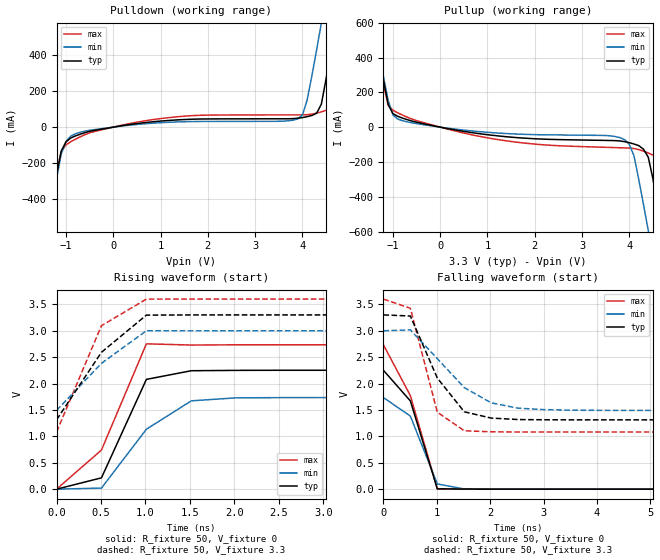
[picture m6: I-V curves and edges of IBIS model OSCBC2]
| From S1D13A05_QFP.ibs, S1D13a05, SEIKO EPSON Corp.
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[Model]   OSCBC2
Model_type Output
Polarity Non-Inverting
Vref=0
Vmeas=1.65
Rref=500
Cref=100pf
C_comp   5p   4p   6p
[Temperature Range] 25   85   -40
[Voltage Range]   3.3   3.0   3.6
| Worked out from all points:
|   slope of the pulldown table from 0 to 0.495 V, typ, clamps not added: 25.1 ohm
|   slope of the pullup table from 0 to 0.495 V, typ, clamps not added: 20.5 ohm
|   falling waveform, R_fixture 50, V_fixture 0: 20-80 % time 484ps typ, 413ps min, 569ps max; typ from 2.25 V to 0 V
|   falling waveform, R_fixture 50, V_fixture 3.3: 20-80 % time 654ps typ, 943ps min, 387ps max; typ from 3.3 V to 1.31 V
|   rising waveform, R_fixture 50, V_fixture 0: 20-80 % time 366ps typ, 594ps min, 495ps max; typ from 0 V to 2.25 V
|   rising waveform, R_fixture 50, V_fixture 3.3: 20-80 % time 571ps typ, 592ps min, 379ps max; typ from 1.31 V to 3.3 V
[Pullup]
-3.3V     3.803A     3.433A     4.322A
-1.4V     601.4mA    587mA      625.7mA
-1.1V     130.5mA    156.1mA    126mA
-1V       78.1mA     71.1mA     97.39mA
-800mV    52.34mA    37.3mA     69.74mA
1.3V      -52.46mA   -35.26mA   -74.72mA
3.9V      -83.39mA   -71.99mA   -119.2mA
4.1V      -96.85mA   -165.8mA   -123mA
4.4V      -172mA     -592.1mA   -148.5mA
4.7V      -625.6mA   -1.039A    -210.9mA
5V        -1.131A    -1.486A    -681.8mA
6.6V      -3.842A    -3.886A    -3.847A
[Pulldown]
-3.3V     -3.817A    -3.425A    -4.397A
-1.4V     -597.9mA   -579.9mA   -635.2mA
-1.1V     -132.9mA   -149.9mA   -136.9mA
-1V       -82.63mA   -79.17mA   -98.77mA
-800mV    -48.94mA   -36.59mA   -67.33mA
1.2V      37.79mA    27.39mA    53.82mA
3.9V      49.68mA    45.38mA    68.43mA
4.1V      58.49mA    151.6mA    69.41mA
4.4V      127.9mA    579.5mA    85.11mA
4.7V      596.4mA    1.026A     130.5mA
5V        1.1A       1.473A     625.9mA
6.6V      3.792A     3.866A     3.738A
[Falling Waveform]
R_fixture=50
V_fixture=0
V_fixture_min=0
V_fixture_max=0
0s        2.252V     1.734V     2.734V
505.1ps   1.671V     1.384V     1.772V
1.01ns    6.165mV    99.37mV    8.891mV
1.515ns   2.162mV    3.244mV    146.9uV
2.02ns    366.3uV    1.402mV    54.15uV
50ns      2.948uV    -22.65uV   18.26uV
[Falling Waveform]
R_fixture=50
V_fixture=3.3
V_fixture_min=3.0
V_fixture_max=3.6
0s        3.3V       3V         3.6V
505.1ps   3.279V     3.016V     3.426V
1.01ns    2.104V     2.471V     1.457V
1.515ns   1.465V     1.924V     1.106V
2.02ns    1.346V     1.634V     1.086V
2.525ns   1.319V     1.534V     1.082V
3.03ns    1.314V     1.505V     1.082V
3.535ns   1.313V     1.495V     1.082V
50ns      1.313V     1.491V     1.083V
[Rising Waveform]
R_fixture=50
V_fixture=0
V_fixture_min=0
V_fixture_max=0
0s        0V         0V         0V
505.1ps   214.2mV    20.52mV    740.8mV
1.01ns    2.079V     1.135V     2.752V
1.515ns   2.243V     1.673V     2.729V
2.02ns    2.25V      1.73V      2.734V
50ns      2.252V     1.734V     2.734V
[Rising Waveform]
R_fixture=50
V_fixture=3.3
V_fixture_min=3.0
V_fixture_max=3.6
0s        1.313V     1.491V     1.082V
505.1ps   2.592V     2.383V     3.096V
1.01ns    3.296V     3.001V     3.599V
50ns      3.3V       3V         3.6V
[Ramp]
R_load=50
dV/dt_r   1.351E+0/3.554E-10   1.041E+0/4.801E-10   1.640E+0/2.744E-10
dV/dt_f   1.192E+0/5.546E-10   9.054E-1/8.133E-10   1.510E+0/3.653E-10
